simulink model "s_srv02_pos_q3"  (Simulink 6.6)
settings: Solver=ode4  StartTime=0.0  StopTime=5  FixedStep=0.002  RelTol=1e-3  AbsTol=1e-6
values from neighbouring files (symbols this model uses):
  IMAX_AMP = 0    [config_srv02.m]
  K = Am / Beq_v    [d_model_param.m]    (also in setup_srv02_exp01_mdl.m = 1)
  ki = -( -AmpMax + kp * e_ss ) / ti / e_ss    [d_i_design.m]    (also in setup_srv02_exp02_pos.m = 0; d_pi_design.m = wn^2*tau/K; setup_srv02_exp03_spd.m = 0)
  kp = wn^2/K*tau    [d_pv_design.m]    (also in setup_srv02_exp02_pos.m = 0; d_pi_design.m = (-1+2*zeta*wn*tau)/K; setup_srv02_exp03_spd.m = 0)
  kv = (-1+2*zeta*wn*tau)/K    [d_pv_design.m]    (also in setup_srv02_exp02_pos.m = 0)
  VMAX_DAC = 10    [setup_srv02_exp02_pos.m]    (also in setup_srv02_exp01_mdl.m; setup_srv02_exp03_spd.m)
  wcf = 2 * pi * 50.0    (= 314.159265359)    [setup_srv02_exp02_pos.m]    (also in setup_srv02_exp03_spd.m)
  zetaf = 0.9    [setup_srv02_exp02_pos.m]    (also in setup_srv02_exp03_spd.m)
undefined symbols (not defined in the file or in its folder): square
libraries: simulink x1

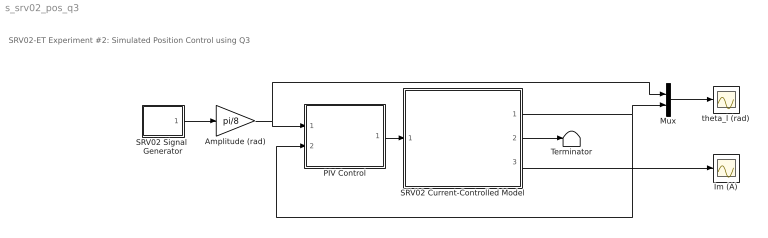
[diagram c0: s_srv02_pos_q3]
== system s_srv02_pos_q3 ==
  note: SRV02-ET Experiment #2: Simulated Position Control using Q3
  Amplitude (rad) : Gain  Gain=pi/8
  Im (A) : Scope
  Mux : Mux  Inputs=2
  PIV Control : Subsystem
  SRV02 Current-Controlled Model : Subsystem
  SRV02 Signal  Generator : Subsystem  mask(QET Signal Generator){sig_type=square, a=1, f=0.4}
      mask prompts: sig_type "Signal Type"; a "Amplitude"; f "Frequency (Hz)"
      mask help: Generates a square, triangular, or sinusoidal waveform of a specified amplitude and frequency.
  Terminator : Terminator
  theta_l (rad) : Scope
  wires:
  SRV02 Current-Controlled Model/2(omega_l (rad/s)) -> Terminator/1
  PIV Control/1(u (A)) -> SRV02 Current-Controlled Model/1(I_ref (A))
  SRV02 Current-Controlled Model/1(theta_l (rad)) -> Mux/2, PIV Control/2(theta_l (rad))
  SRV02 Current-Controlled Model/3(Im (A)) -> Im (A)/1
  Mux/1 -> theta_l (rad)/1
  SRV02 Signal  Generator/1(out) -> Amplitude (rad)/1
  Amplitude (rad)/1 -> PIV Control/1(theta_d (rad)), Mux/1

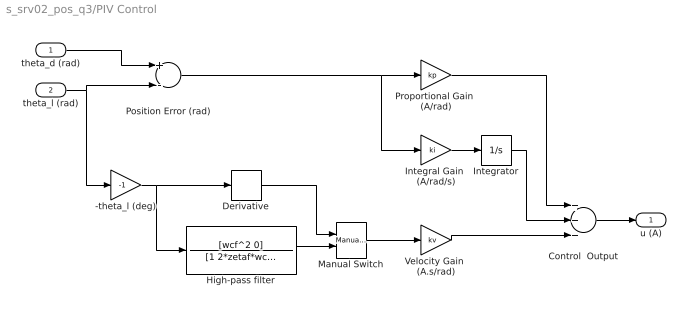
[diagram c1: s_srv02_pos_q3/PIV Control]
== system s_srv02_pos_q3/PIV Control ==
  theta_d (rad) : Inport
  theta_l (rad) : Inport  Port=2
  -theta_l (deg) : Gain  Gain=-1
  Control  Output : Sum  Inputs=+++  OutScaling=2^-10
  Derivative : Derivative
  High-pass filter : TransferFcn  Numerator=[wcf^2 0]  Denominator=[1 2*zetaf*wcf wcf^2]
  Integral Gain  (A/rad/s) : Gain  Gain=ki
  Integrator : Integrator
  Manual Switch : simulink/Signal Routing/Manual Switch  SystemSampleTime=-1  sw=0  action=0  varsize=off
  Position Error (rad) : Sum  Inputs=+-  OutScaling=2^-10
  Proportional Gain  (A/rad) : Gain  Gain=kp
  Velocity Gain  (A.s/rad) : Gain  Gain=kv
  u (A) : Outport
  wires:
  Proportional Gain  (A/rad)/1 -> Control  Output/1
  theta_d (rad)/1 -> Position Error (rad)/1
  Control  Output/1 -> u (A)/1
  theta_l (rad)/1 -> Position Error (rad)/2, -theta_l (deg)/1
  Position Error (rad)/1 -> Proportional Gain  (A/rad)/1, Integral Gain  (A/rad/s)/1
  -theta_l (deg)/1 -> Derivative/1, High-pass filter/1
  High-pass filter/1 -> Manual Switch/2
  Manual Switch/1 -> Velocity Gain  (A.s/rad)/1
  Derivative/1 -> Manual Switch/1
  Integral Gain  (A/rad/s)/1 -> Integrator/1
  Velocity Gain  (A.s/rad)/1 -> Control  Output/3
  Integrator/1 -> Control  Output/2

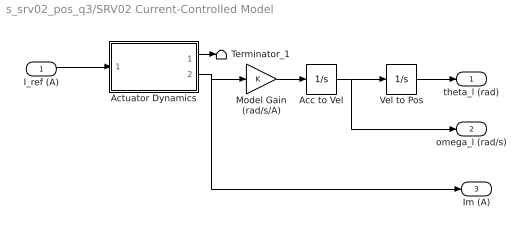
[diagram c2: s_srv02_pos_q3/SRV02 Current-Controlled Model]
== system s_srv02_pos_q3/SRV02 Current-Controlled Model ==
  I_ref (A) : Inport
  Acc to Vel : Integrator
  Actuator Dynamics : Subsystem
  Model Gain (rad/s/A) : Gain  Gain=K
  Terminator_1 : Terminator
  Vel to Pos : Integrator
  theta_l (rad) : Outport
  omega_l (rad/s) : Outport  Port=2
  Im (A) : Outport  Port=3
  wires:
  Vel to Pos/1 -> theta_l (rad)/1
  Actuator Dynamics/2(Im (A)) -> Im (A)/1, Model Gain (rad/s/A)/1
  I_ref (A)/1 -> Actuator Dynamics/1(I_ref (A))
  Actuator Dynamics/1(Vdaq (V)) -> Terminator_1/1
  Model Gain (rad/s/A)/1 -> Acc to Vel/1
  Acc to Vel/1 -> Vel to Pos/1, omega_l (rad/s)/1

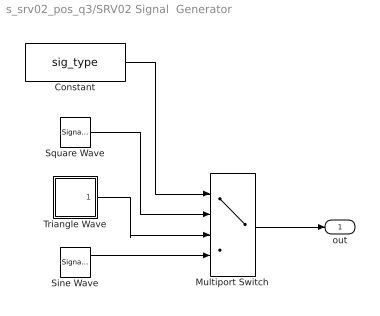
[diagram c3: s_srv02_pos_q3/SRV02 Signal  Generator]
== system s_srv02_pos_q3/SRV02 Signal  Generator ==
  Constant : Constant  Value=sig_type
  Multiport Switch : MultiPortSwitch  Inputs=3
  Sine Wave : SignalGenerator  Amplitude=a  Frequency=f
  Square Wave : SignalGenerator  WaveForm=square  Amplitude=a  Frequency=f
  Triangle Wave : Subsystem
  out : Outport
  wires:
  Square Wave/1 -> Multiport Switch/2
  Triangle Wave/1(out) -> Multiport Switch/3
  Sine Wave/1 -> Multiport Switch/4
  Multiport Switch/1 -> out/1
  Constant/1 -> Multiport Switch/1

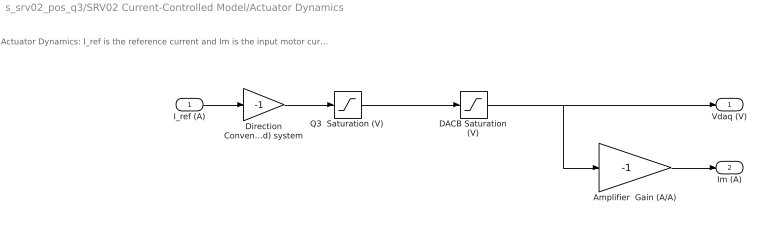
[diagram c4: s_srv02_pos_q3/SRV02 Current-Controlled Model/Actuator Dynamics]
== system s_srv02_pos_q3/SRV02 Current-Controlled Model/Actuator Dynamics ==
  note: Actuator Dynamics: I_ref is the reference current and Im is the input motor current after going through the DACB and amplifier limitiations.
  I_ref (A) : Inport
  Amplifier  Gain (A/A) : Gain  Gain=-1
  DACB Saturation (V) : Saturate  UpperLimit=VMAX_DAC  LowerLimit=-VMAX_DAC
  Direction Convention: (Right-Hand) system : Gain  Gain=-1
  Q3  Saturation (V) : Saturate  UpperLimit=IMAX_AMP  LowerLimit=-IMAX_AMP
  Vdaq (V) : Outport
  Im (A) : Outport  Port=2
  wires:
  Direction Convention: (Right-Hand) system/1 -> Q3  Saturation (V)/1
  Amplifier  Gain (A/A)/1 -> Im (A)/1
  DACB Saturation (V)/1 -> Vdaq (V)/1, Amplifier  Gain (A/A)/1
  Q3  Saturation (V)/1 -> DACB Saturation (V)/1
  I_ref (A)/1 -> Direction Convention: (Right-Hand) system/1

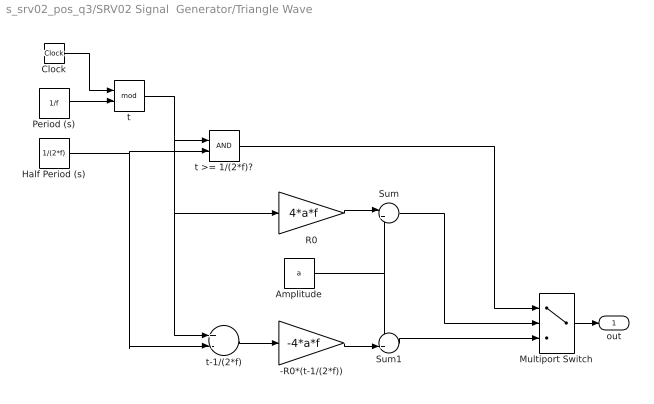
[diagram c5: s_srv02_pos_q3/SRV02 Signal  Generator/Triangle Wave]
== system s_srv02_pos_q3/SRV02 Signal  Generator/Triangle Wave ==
  -R0*(t-1/(2*f)) : Gain  Gain=-4*a*f
  Amplitude : Constant  Value=a
  Clock : Clock
  Half Period (s) : Constant  Value=1/(2*f)
  Multiport Switch : MultiPortSwitch  Inputs=2  zeroidx=on
  Period (s) : Constant  Value=1/f
  R0 : Gain  Gain=4*a*f
  Sum : Sum  Inputs=|+-
  Sum1 : Sum  Inputs=++|
  t : Math  Operator=mod
  t >= 1/(2*f)? : RelationalOperator  LogicOutDataTypeMode=Boolean
  t-1/(2*f) : Sum  Inputs=+-  OutScaling=2^-10
  out : Outport
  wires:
  Sum1/1 -> Multiport Switch/3
  Sum/1 -> Multiport Switch/2
  t >= 1/(2*f)?/1 -> Multiport Switch/1
  -R0*(t-1/(2*f))/1 -> Sum1/2
  Amplitude/1 -> Sum1/1, Sum/2
  R0/1 -> Sum/1
  t-1/(2*f)/1 -> -R0*(t-1/(2*f))/1
  Half Period (s)/1 -> t-1/(2*f)/2, t >= 1/(2*f)?/2
  t/1 -> t-1/(2*f)/1, R0/1, t >= 1/(2*f)?/1
  Period (s)/1 -> t/2
  Clock/1 -> t/1
  Multiport Switch/1 -> out/1
